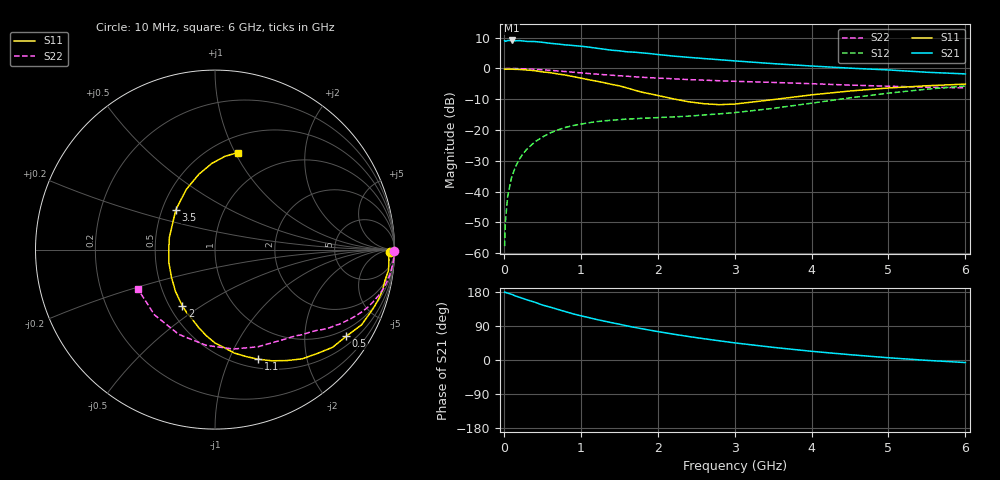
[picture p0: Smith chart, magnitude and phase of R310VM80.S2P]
! SIEMENS Small Signal Semiconductors
! BFR181
! Si NPN RF Bipolar Junction Transistor in SOT23
! VCE = 10 V  IC = 0.8 mA
! Common Emitter S-Parameters:  May  1996
# GHz  S  MA  R  50
!  f  S11  S21  S12  S22
! GHz  MAG  ANG  MAG  ANG  MAG  ANG  MAG  ANG
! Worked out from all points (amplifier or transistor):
!   36 points, 10 MHz to 6 GHz, reference 50 ohm
!   highest |S21| = 9.1 dB at 100 MHz (marker M1)
!   |S21| within 3 dB of that: start of sweep to 1.352 GHz
!   unconditionally stable (mu >= 1): 2.201 GHz to 3.802 GHz
!   at 250 MHz: K = 0.14, MSG = 18.3 dB, |S12| = -27.7 dB
!   at 1.4 GHz: K = 0.69, MSG = 11.4 dB, |S12| = -16.9 dB
!   at 6 GHz: K = 0.88, MSG = 2.0 dB, |S12| = -5.7 dB
!   S11 on the Smith chart (normalised r, x): 10 MHz: 57, -36; 500 MHz: 0.76, -3.17; 1.1 GHz: 0.60, -1.28; 2 GHz: 0.58, -0.42; 3.5 GHz: 0.59, +0.29; 6 GHz: 0.66, +1.03
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0.01  0.9754 -0.9  2.819 179.2  0.0013 88.6  0.9984 -0.4
0.02  0.967 -1.4  2.748 178.4  0.0032 81.7  0.9889 -0.6
0.05  0.9712 -3.4  2.829 176.5  0.0084 87.1  0.9977 -1.6
0.1  0.9736 -6.8  2.839 173.4  0.0168 85.8  0.9971 -3.2
0.15  0.9628 -10.1  2.799 169.1  0.025 83.2  0.9926 -5.0
0.2  0.9608 -13.5  2.825 165.8  0.0333 80.5  0.9888 -6.6
0.25  0.9522 -16.9  2.79 162.3  0.0412 78.1  0.9847 -8.2
0.4  0.9179 -27.2  2.727 152.7  0.0636 72.3  0.9651 -12.7
0.5  0.8763 -33.4  2.652 145.2  0.0765 68.3  0.9474 -15.6
0.7  0.8126 -45.4  2.486 133.7  0.1001 60.8  0.909 -20.8
0.9  0.737 -57.0  2.352 121.8  0.1181 54.8  0.8673 -25.2
1.1  0.6559 -68.6  2.218 112.1  0.1307 50.0  0.8252 -29.2
1.3  0.5865 -79.4  2.051 102.9  0.1407 46.4  0.7903 -32.4
1.6  0.4821 -95.8  1.858 90.0  0.1505 42.8  0.747 -36.6
1.8  0.4095 -107.8  1.785 82.3  0.1548 42.1  0.7173 -39.1
2  0.3636 -119.9  1.679 75.0  0.159 41.7  0.6965 -41.6
2.2  0.3208 -133.3  1.585 68.4  0.1629 41.9  0.6783 -44.4
2.8  0.2576 -179.6  1.383 50.7  0.1827 45.9  0.6301 -52.7
3.5  0.3111 134.6  1.194 33.4  0.2245 49.8  0.5919 -66.2
4.5  0.4293 102.1  1.008 14.0  0.3324 48.1  0.5355 -95.4
5.5  0.5221 84.0  0.865 -1.0  0.4595 36.5  0.4959 -132.9
6  0.5555 76.8  0.813 -6.7  0.5179 28.5  0.4823 -152.9
